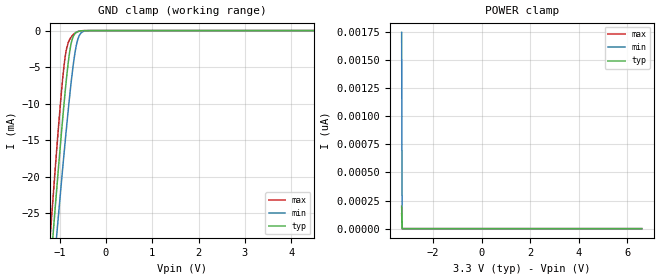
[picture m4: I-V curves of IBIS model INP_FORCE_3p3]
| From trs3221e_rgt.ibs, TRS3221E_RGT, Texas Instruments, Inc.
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[Model]   INP_FORCE_3p3
Model_type   Input
Vinl = 0.8
Vinh = 2
|   typ   min   max
C_comp   0.802pF	0.773pF	0.843pF
[Voltage Range]   3.3   3   3.6
[Temperature Range]   27   110   -40
[Power Clamp Reference]   3.3   3   3.6
[GND Clamp Reference]   0   0   0
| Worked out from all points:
|   GND clamp passes 1 mA (typ) near -0.72 V on its own axis
[GND Clamp]
|   Voltage   I(typ)   I(min)   I(max)
-3.3V     -208.9mA   -199.9mA   -218.1mA
-1.191V   -31.96mA   -37.48mA   -27.18mA
-1.092V   -24.11mA   -30.22mA   -18.8mA
-1.023V   -18.75mA   -25.23mA   -13.19mA
-943.8mV  -12.86mA   -19.64mA   -7.328mA
-884.4mV  -8.728mA   -15.57mA   -3.85mA
-815.1mV  -4.523mA   -11.03mA   -1.689mA
-755.7mV  -1.958mA   -7.437mA   -943.5uA
-627mV    -207.2uA   -1.704mA   -193.8uA
-547.8mV  -50.69uA   -415.8uA   -45.78uA
-399.3mV  -2.68uA    -15.23uA   -1.444uA
6.6V      0A         0A         0A
[POWER Clamp]
|   Voltage   I(typ)   I(min)   I(max)
-3.3V     199.5pA    1.746nA    133.2pA
-3.28V    0A         0A         0A
-3.27V    0A         0A         0A
6.6V      0A         0A         0A
